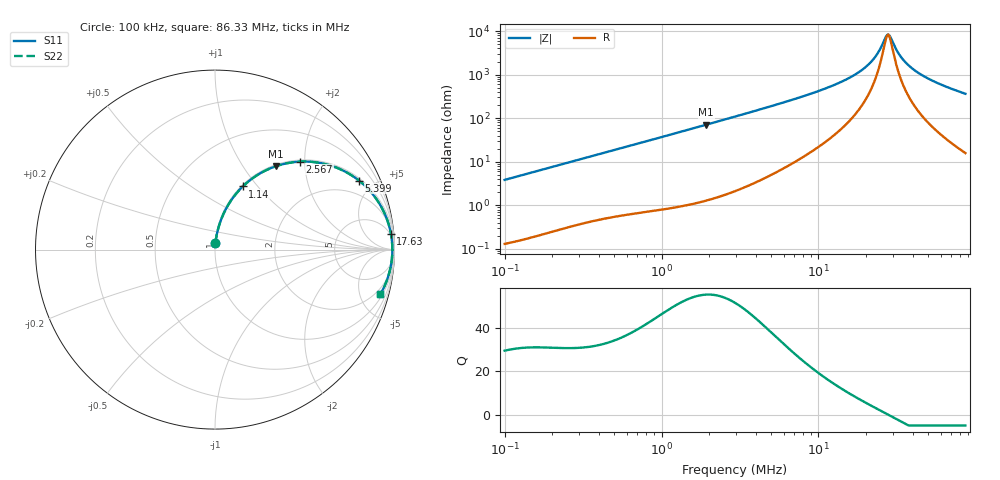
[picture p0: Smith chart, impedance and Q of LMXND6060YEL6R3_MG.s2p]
! LMXND6060YEL6R3_MG  S-PARAMETER MODEL  ( General Type )
! Model Generated by TAIYO YUDEN Corporation (https://www.yuden.co.jp/en/)
! Version 1.0
! TAIYO YUDEN Control No. 191025NI43SB-FBB
! Copyright(c) 2019 TAIYO YUDEN CO.,LTD. All Rights Reserved.
! Product Description (link to TY-COMPAS)
! https://ds.yuden.co.jp/TYCOMPAS/or/detail?pn=LMXND6060YEL6R3MMG&u=M
! Products Name : Inductors
! Characteristics :
!  Inductance : 6.3 uH , SRF(min) : 15 MHz , DC Resistance(max) : 0.0468 Ohm
!  Rated Current : Saturation :3600 mA , Temp Rise : 3000 mA (40 degC)
!  Case Size : 6.0 x 6.0 / 0.236 x 0.236 [mm/inch] , Thickness : 4.5 / 0.177 [mm/inch]
!  (Conditions: Temperature = 25 degC , DC Bias Current/Voltage = 0A / 0V)
! External Node Assignments :
!  1  o---GGG---o  2
! GND o---------o GND
! Frequency Range : 0.1MHz  -  86.325287MHz  [ 402 STEP ]
# MHz S RI R 50
! Freq[MHz].  S11 Real  S11 Imag  S21 Real  S21 Imag  S12 Real  S12 Imag  S22 Real  S22 Imag
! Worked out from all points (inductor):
!   401 points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, 100 kHz to 86.33 MHz, reference 50 ohm
!   read as one part in series: L = 6.09 uH near 103.4 kHz
!   highest Q = 55.2 at 1.926 MHz (marker M1), where L = 5.86 uH
!   self-resonance near 27.35 MHz
!   S11 on the Smith chart (normalised r, x): 100 kHz: 1.00, +0.08; 1.14 MHz: 1.02, +0.84; 2.567 MHz: 1.04, +1.90; 5.399 MHz: 1.12, +4.11; 17.63 MHz: 4, +21; 86.33 MHz: 1.32, -7.28
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0.1  0.00277 0.0382  0.9972 -0.0382  0.9972 -0.0382  0.00277 0.0382
0.310315  0.0171 0.1143  0.9829 -0.1143  0.9829 -0.1143  0.0171 0.1143
0.599897  0.0523 0.2095  0.9477 -0.2095  0.9477 -0.2095  0.0523 0.2095
0.962956  0.1172 0.3109  0.8828 -0.3109  0.8828 -0.3109  0.1172 0.3109
1.140275  0.155 0.3518  0.845 -0.3518  0.845 -0.3518  0.155 0.3518
1.925575  0.3376 0.4639  0.6624 -0.4639  0.6624 -0.4639  0.3376 0.4639
2.566529  0.4741 0.4901  0.5259 -0.4901  0.5259 -0.4901  0.4741 0.4901
2.938117  0.5415 0.4887  0.4585 -0.4887  0.4585 -0.4887  0.5415 0.4887
5.399101  0.8018 0.3849  0.1982 -0.3849  0.1982 -0.3849  0.8018 0.3849
9.117424  0.9233 0.2437  0.0767 -0.2437  0.0767 -0.2437  0.9233 0.2437
13.44931  0.9652 0.1482  0.0348 -0.1482  0.0348 -0.1482  0.9652 0.1482
17.62567  0.9799 0.0895  0.0201 -0.0895  0.0201 -0.0895  0.9799 0.0895
21.95685  0.986 0.0454  0.014 -0.0454  0.014 -0.0454  0.986 0.0454
24.30033  0.9875 0.0256  0.0125 -0.0256  0.0125 -0.0256  0.9875 0.0256
26.89393  0.9881 0.00609  0.0119 -0.00609  0.0119 -0.00609  0.9881 0.00609
27.81858  0.9882 -0.000402  0.0118 0.000402  0.0118 0.000402  0.9882 -0.000402
28.29276  0.9882 -0.00365  0.0118 0.00365  0.0118 0.00365  0.9882 -0.00365
33.50261  0.9869 -0.0363  0.0131 0.0363  0.0131 0.0363  0.9869 -0.0363
36.45696  0.9854 -0.0529  0.0146 0.0529  0.0146 0.0529  0.9854 -0.0529
40.34805  0.9828 -0.0731  0.0172 0.0731  0.0172 0.0731  0.9828 -0.0731
55.62744  0.9675 -0.1415  0.0325 0.1415  0.0325 0.1415  0.9675 -0.1415
86.32529  0.9206 -0.2495  0.0794 0.2495  0.0794 0.2495  0.9206 -0.2495
